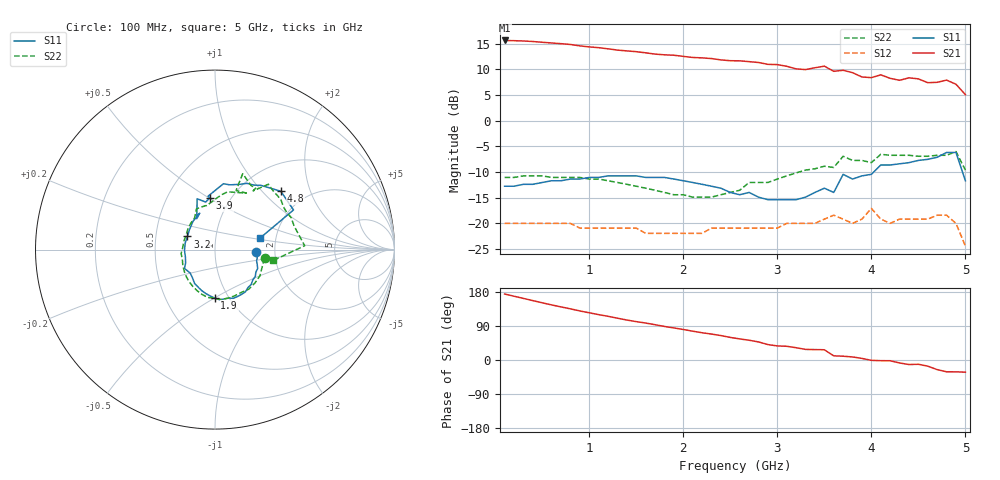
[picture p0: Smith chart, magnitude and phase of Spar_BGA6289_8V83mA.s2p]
!BGA6289
!Scattering parameters
!Is=83mA Vs=8V
!Pd=-30dBm
!Z0=50 Ohm
!Tamb 25C
#  MHz  S  MA  R 50
! Freq  S11  S21  S12  S22  :
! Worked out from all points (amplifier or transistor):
!   50 points, 100 MHz to 5 GHz, reference 50 ohm
!   highest |S21| = 15.6 dB at 100 MHz (marker M1)
!   |S21| within 3 dB of that: start of sweep to 1.955 GHz
!   unconditionally stable (mu >= 1): start of sweep to end of sweep
!   at 900 MHz: K = 1.17, MAG = 15.3 dB, |S12| = -20.9 dB
!   at 2.6 GHz: K = 1.49, MAG = 12.1 dB, |S12| = -20.9 dB
!   at 5 GHz: K = 3.85, MAG = 6.0 dB, |S12| = -24.4 dB
!   S11 on the Smith chart (normalised r, x): 100 MHz: 1.59, -0.05; 1.9 GHz: 0.86, -0.50; 3.2 GHz: 0.73, +0.11; 3.9 GHz: 0.80, +0.51; 4.8 GHz: 1.50, +1.28; 5 GHz: 1.65, +0.23
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100  0.23 -3.6  6.03 174.1  0.1 -1.6  0.28 -9.9
300  0.24 -10.7  5.96 162.6  0.1 -5.0  0.29 -30.4
600  0.26 -23.9  5.7 145.4  0.1 -9.4  0.28 -58.5
1000  0.28 -43.8  5.22 124.6  0.09 -12.5  0.27 -91.0
1400  0.29 -64.2  4.77 105.5  0.09 -13.9  0.24 -120.7
1800  0.28 -85.1  4.37 88.5  0.08 -13.1  0.2 -153.6
1900  0.27 -90.4  4.33 84.6  0.08 -12.9  0.19 -163.2
2600  0.19 -137.0  3.82 55.6  0.09 -10.4  0.21 122.8
3000  0.17 -178.5  3.51 37.1  0.09 -10.9  0.27 92.7
3200  0.17 154.5  3.19 32.4  0.1 -9.9  0.31 82.5
3400  0.2 127.7  3.27 27.5  0.1 -8.6  0.34 69.3
3500  0.22 112.8  3.39 27.0  0.11 -7.7  0.36 61.0
3600  0.2 120.6  3.02 11.0  0.12 -15.4  0.35 70.4
3700  0.3 109.3  3.09 10.0  0.11 -29.9  0.45 69.9
3900  0.29 95.5  2.66 4.2  0.11 -18.1  0.41 56.5
4100  0.37 82.7  2.79 -1.8  0.11 -32.9  0.47 50.8
4200  0.37 77.1  2.58 -1.9  0.1 -29.1  0.46 44.8
4400  0.39 68.9  2.61 -12.0  0.11 -26.3  0.46 36.9
4500  0.41 64.2  2.55 -11.3  0.11 -27.4  0.45 32.1
4600  0.42 58.8  2.34 -16.2  0.11 -29.9  0.45 27.3
4800  0.49 41.6  2.48 -31.1  0.12 -30.8  0.46 16.6
5000  0.26 14.4  1.79 -32.1  0.06 1.0  0.33 -10.6
